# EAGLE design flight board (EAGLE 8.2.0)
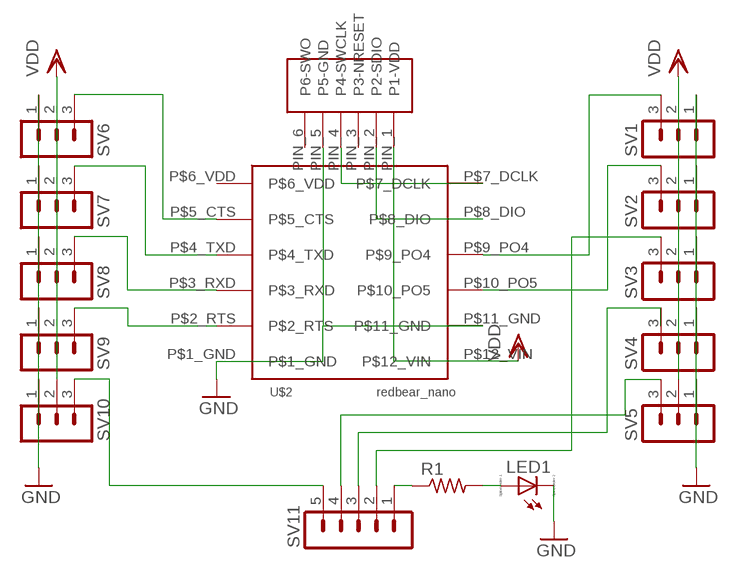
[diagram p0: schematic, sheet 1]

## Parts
LED1  LED_ESML0603  [LED_SML0603]
R1  R-US_R0603  [R0603]
SV1  MA03-1  [MA03-1]
SV2  MA03-1  [MA03-1]
SV3  MA03-1  [MA03-1]
SV4  MA03-1  [MA03-1]
SV5  MA03-1  [MA03-1]
SV6  MA03-1  [MA03-1]
SV7  MA03-1  [MA03-1]
SV8  MA03-1  [MA03-1]
SV9  MA03-1  [MA03-1]
SV10  MA03-1  [MA03-1]
SV11  MA05-1  [MA05-1]
U$1  TAG_CONNCET  [TAG_CONNECT]
U$2  REDBEAR_NANO  [REDBEAR_NANO]

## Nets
GND: LED1.C SV1.1 SV2.1 SV3.1 SV4.1 SV5.1 SV6.1 SV7.1 SV8.1 SV9.1 SV10.1 U$1.PIN_5(P5-GND) U$2.P$1_GND U$2.P$11_GND
N$1: SV6.3 U$2.P$5_CTS
N$2: SV7.3 U$2.P$4_TXD
N$3: U$1.PIN_4(P4-SWCLK) U$2.P$7_DCLK
N$4: U$1.PIN_2(P2-SDIO) U$2.P$8_DIO
N$5: SV8.3 U$2.P$3_RXD
N$6: SV9.3 U$2.P$2_RTS
N$7: SV10.3 SV11.5
N$8: R1.1 SV11.1
N$9: SV1.3 U$2.P$9_PO4
N$10: SV2.3 U$2.P$10_PO5
N$11: SV5.3 SV11.4
N$12: SV4.3 SV11.3
N$13: LED1.A R1.2
N$14: SV3.3 SV11.2
VDD: SV1.2 SV2.2 SV3.2 SV4.2 SV5.2 SV6.2 SV7.2 SV8.2 SV9.2 SV10.2 U$1.PIN_1(P1-VDD) U$2.P$12_VIN
Unconnected: U$1.PIN_3(P3-NRESET) U$1.PIN_6(P6-SWO) U$2.P$6_VDD

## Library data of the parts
LED1 = eagle-ltspice:LED_E: LED; SPICEMODEL: NONE; SPICEPREFIX: D; SPICETYPE: diode
R1 = resistor:R-US_: RESISTOR, American symbol
SV1-SV10 = con-lstb:MA03-1: PIN HEADER; OC_FARNELL: unknown; OC_NEWARK: unknown
SV11 = con-lstb:MA05-1: PIN HEADER; OC_FARNELL: unknown; OC_NEWARK: unknown
U$1 = tag_connect:TAG_CONNCET
U$2 = redbearnano:REDBEAR_NANO

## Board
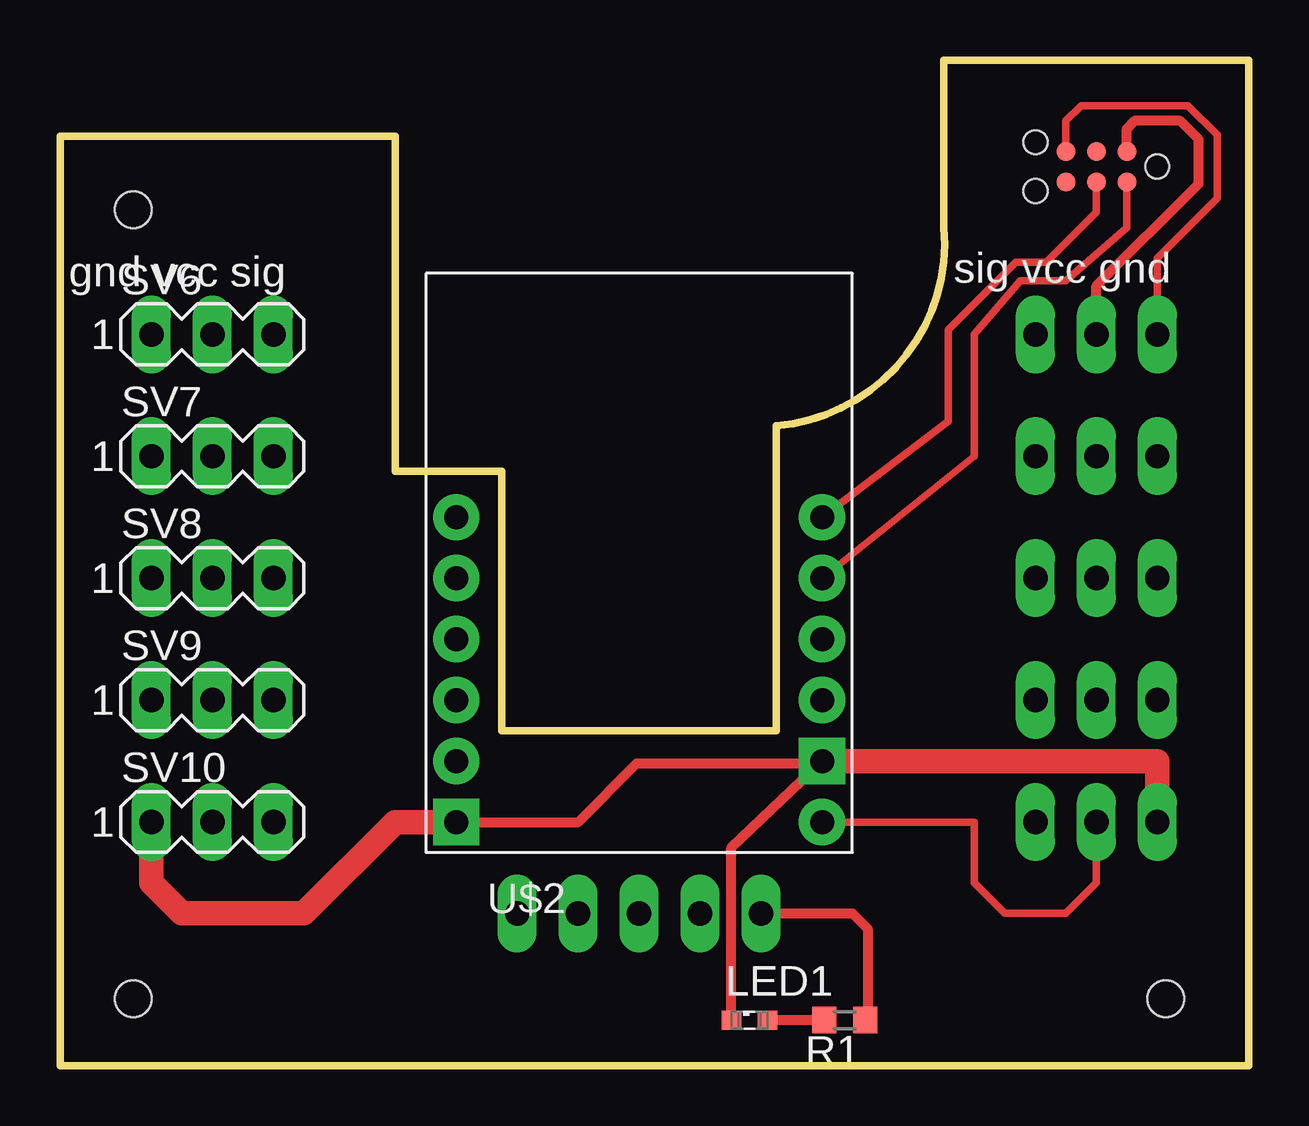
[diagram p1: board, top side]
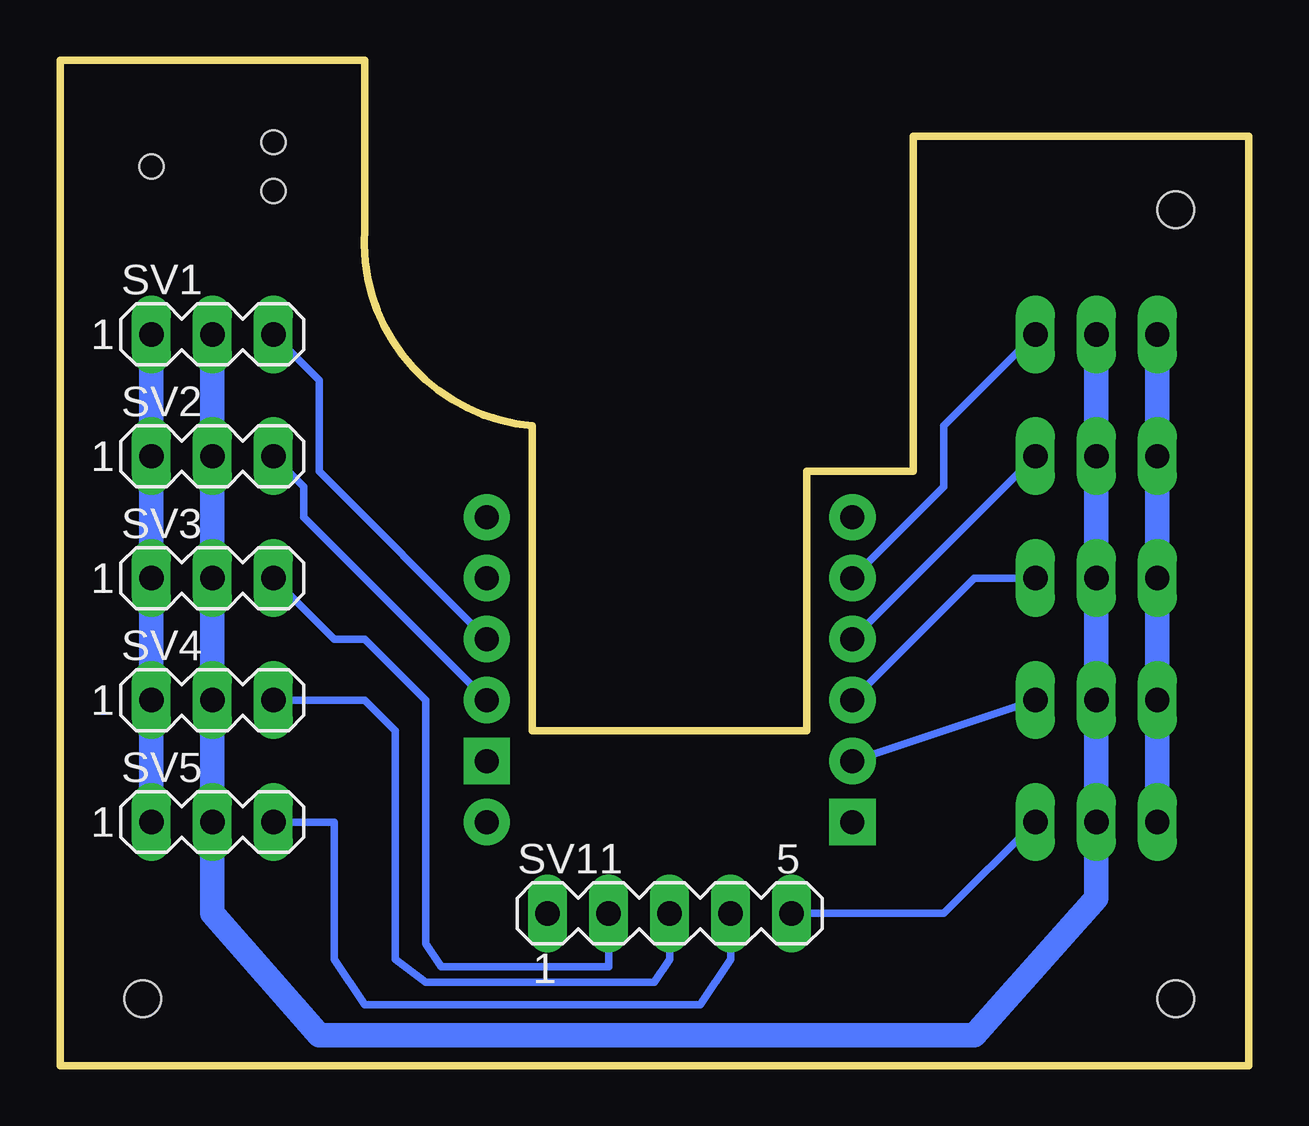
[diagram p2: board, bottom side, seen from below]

Size 49.53 x 41.91 mm. Coordinates in mm from the lower left corner, seen from the top.
Outline: 0,38.73 13.97,38.73 13.97,24.76 18.41,24.76 18.41,13.97 29.85,13.97 29.85,26.67 arc90 36.83,34.92 36.83,41.91 49.53,41.91 49.53,0 0,0 0,38.73
Copper layers (1*16): Top 0.035mm / dielectric 1.5mm / Bottom 0.035mm
Design rules "SparkFun": minimum track width 8mil, minimum drill 20mil, track to track 8mil, track to pad 8mil, pad to pad 8mil, via to via 8mil, smd to smd 8mil, copper to edge 8mil, drill to drill 8mil, minimum pad ring 12mil, minimum via ring 10mil, stop-mask expansion 4mil, vias tented up to drill 20mil, thermal gap 10mil
Holes 1.52 mm at 3.05,35.66 3.05,2.79 46.08,2.79

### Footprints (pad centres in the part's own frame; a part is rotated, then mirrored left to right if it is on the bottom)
LED_SML0603 = smd 0.8 x 0.8: A 0.75,0; C -0.75,0
R0603 = smd 1 x 1.1: 1 -0.85,0; 2 0.85,0
MA03-1 = drill 1.016 long: 1 -2.54,0; 2 0,0; 3 2.54,0
MA05-1 = drill 1.016 long: 1 -5.08,0; 2 -2.54,0; 3 0,0; 4 2.54,0; 5 5.08,0
TAG_CONNECT = smd 0.787 x 0.787: PIN_1 1.27,-0.635; PIN_2 1.27,0.635; PIN_3 2.54,-0.635; PIN_4 2.54,0.635; PIN_5 3.81,-0.635; PIN_6 3.81,0.635 | hole 1: 0,0; 5.08,1.016; 5.08,-1.016
REDBEAR_NANO = drill 1 pad 1.93 square: P$1_GND 0,0; P$11_GND 15.24,2.54 | drill 1 pad 1.93: P$2_RTS 0,2.54; P$3_RXD 0,5.08; P$4_TXD 0,7.62; P$5_CTS 0,10.16; P$6_VDD 0,12.7; P$7_DCLK 15.24,12.7; P$8_DIO 15.24,10.16; P$9_PO4 15.24,7.62; P$10_PO5 15.24,5.08; P$12_VIN 15.24,0

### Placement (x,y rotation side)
LED1  28.73,1.9 0 top
R1  32.7,1.9 180 top
SV1  43.18,30.48 0 bottom
SV2  43.18,25.4 0 bottom
SV3  43.18,20.32 0 bottom
SV4  43.18,15.24 0 bottom
SV5  43.18,10.16 0 bottom
SV6  6.35,30.48 0 top
SV7  6.35,25.4 0 top
SV8  6.35,20.32 0 top
SV9  6.35,15.24 0 top
SV10  6.35,10.16 0 top
SV11  24.13,6.35 0 bottom
U$1  45.72,37.47 180 top
U$2  16.51,10.16 0 top

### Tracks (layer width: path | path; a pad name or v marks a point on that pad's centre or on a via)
GND
  Top 0.305: SV1.1 45.72,33.66 48.21,36.14 48.21,38.79 46.99,40 42.55,40 41.91,39.37 U$1.PIN_5
  Top 0.406: LED1.C 27.98,9.09 U$2.P$11_GND 31.65,12.6 24.03,12.6 21.59,10.16 U$2.P$1_GND
  Top 1.016: U$2.P$1_GND 13.97,10.16 10.16,6.35 5.08,6.35 3.81,7.62 SV10.1 | U$2.P$11_GND 45.72,12.7 SV5.1
  Bottom 1.016: SV1.1 SV2.1 SV3.1 | SV3.1 45.72,19.68 | SV3.1 SV4.1 SV5.1 | SV6.1 SV7.1 SV8.1 | SV8.1 3.81,19.68 | SV8.1 SV9.1 SV10.1
N$1
  Bottom 0.305: U$2.P$5_CTS 12.7,24.13 12.7,26.67 SV6.3
N$2
  Bottom 0.305: U$2.P$4_TXD SV7.3
N$3
  Top 0.305: U$1.PIN_4 43.18,35.56 41.1,33.48 39.82,33.48 37.01,30.67 37.01,26.85 35.7,25.85 U$2.P$7_DCLK
N$4
  Top 0.305: U$2.P$8_DIO 38.1,25.4 38.1,30.48 40,32.7 41.91,32.7 44.45,34.92 U$1.PIN_2
N$5
  Bottom 0.305: SV8.3 11.43,20.32 U$2.P$3_RXD
N$6
  Bottom 0.305: U$2.P$2_RTS SV9.3
N$7
  Bottom 0.305: SV11.5 12.7,6.35 SV10.3
N$8
  Top 0.406: SV11.1 33.02,6.35 33.66,5.71 33.66,2.01 R1.1
N$9
  Bottom 0.305: U$2.P$9_PO4 38.73,24.76 38.73,28.57 SV1.3
N$10
  Bottom 0.305: SV2.3 39.37,24.13 39.37,22.86 U$2.P$10_PO5
N$11
  Bottom 0.305: SV5.3 38.1,10.16 38.1,4.45 36.83,2.54 22.86,2.54 21.59,4.45 SV11.4
N$12
  Bottom 0.305: SV4.3 36.83,15.24 35.56,13.97 35.56,4.45 34.29,3.49 24.76,3.49 24.13,4.45 SV11.3
N$13
  Top 0.406: R1.2 LED1.A
N$14
  Bottom 0.305: SV3.3 38.1,17.78 36.83,17.78 34.29,15.24 34.29,5.08 33.66,4.13 26.67,4.13 SV11.2
VDD
  Top 0.305: U$2.P$12_VIN 38.1,10.16 38.1,7.62 39.37,6.35 41.91,6.35 43.18,7.62 SV5.2
  Top 0.406: SV1.2 43.18,32.49 47.44,36.75 47.44,38.6 46.67,39.37 44.77,39.37 44.45,39.05 U$1.PIN_1
  Bottom 1.016: SV1.2 SV2.2 SV3.2 SV4.2 SV5.2 43.18,6.35 38.73,1.27 11.43,1.27 6.35,6.98 SV10.2 SV9.2 SV8.2 SV7.2 SV6.2

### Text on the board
tPlace: gnd vcc sig | sig vcc gnd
